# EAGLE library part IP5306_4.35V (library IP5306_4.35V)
2.1A Charging 2.4 A Discharge Highly Integrated Mobile Power Supply Source: Datasheet
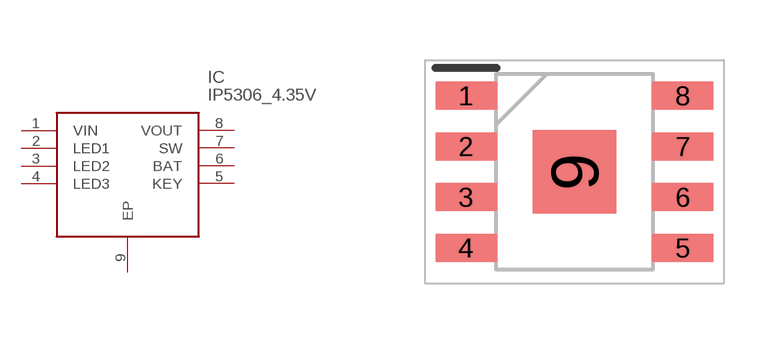
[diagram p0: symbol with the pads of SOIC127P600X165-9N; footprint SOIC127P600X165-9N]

Designator prefix IC

## IP5306_4.35V (Description: 2.1A Charging 2.4 A Discharge Highly Integrated Mobile Power Supply; Height: 1.65mm; Manufacturer_Name: INJOINIC; Manufacturer_Part_Number: IP5306_4.35V)  [SOIC127P600X165-9N]
1  VIN
2  LED1
3  LED2
4  LED3
5  KEY
6  BAT
7  SW
8  VOUT
9  EP

## Footprint SOIC127P600X165-9N (pad centres in mm)
IP5306
smd 1.525 x 0.7: 1 -2.712,1.905; 2 -2.712,0.635; 3 -2.712,-0.635; 4 -2.712,-1.905; 5 2.712,-1.905; 6 2.712,-0.635; 7 2.712,0.635; 8 2.712,1.905
smd 2.09 x 2.09: 9 0,0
